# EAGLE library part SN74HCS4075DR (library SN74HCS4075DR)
Logic Gates 3-channel, 3-input OR gates with schmitt-trigger inputs Source: Datasheet
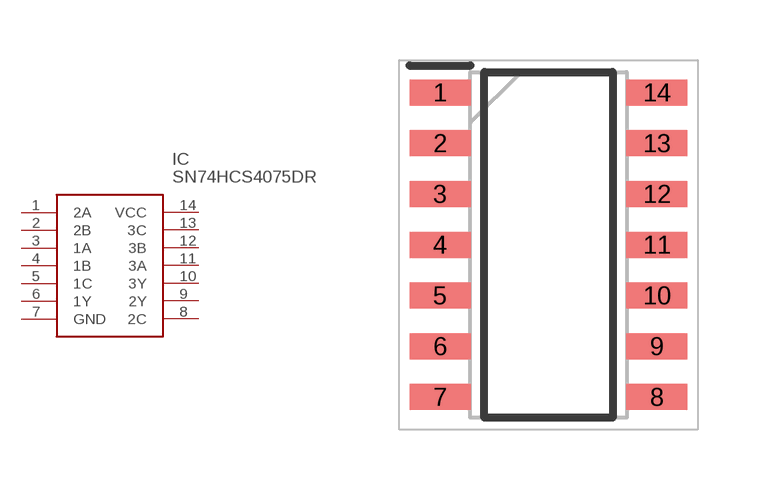
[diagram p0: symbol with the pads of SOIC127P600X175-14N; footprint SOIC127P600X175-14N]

Designator prefix IC

## SN74HCS4075DR (Description: Logic Gates 3-channel, 3-input OR gates with schmitt-trigger inputs; Height: 1.75mm; Manufacturer_Name: Texas Instruments; Manufacturer_Part_Number: SN74HCS4075DR; Mouser_Part_Number: 595-SN74HCS4075DR; Mouser_Price-Stock: https://www.mouser.co.uk/ProductDetail/Texas-Instruments/SN74HCS4075DR?qs=sPbYRqrBIVmdJ91ff%252BdGMg%3D%3D)  [SOIC127P600X175-14N]
1  2A
2  2B
3  1A
4  1B
5  1C
6  1Y
7  GND
8  2C
9  2Y
10  3Y
11  3A
12  3B
13  3C
14  VCC

## Footprint SOIC127P600X175-14N (pad centres in mm)
D (-R-PDSO-G14)
smd 1.525 x 0.65: 1 -2.712,3.81; 2 -2.712,2.54; 3 -2.712,1.27; 4 -2.712,0; 5 -2.712,-1.27; 6 -2.712,-2.54; 7 -2.712,-3.81; 8 2.712,-3.81; 9 2.712,-2.54; 10 2.712,-1.27; 11 2.712,0; 12 2.712,1.27; 13 2.712,2.54; 14 2.712,3.81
